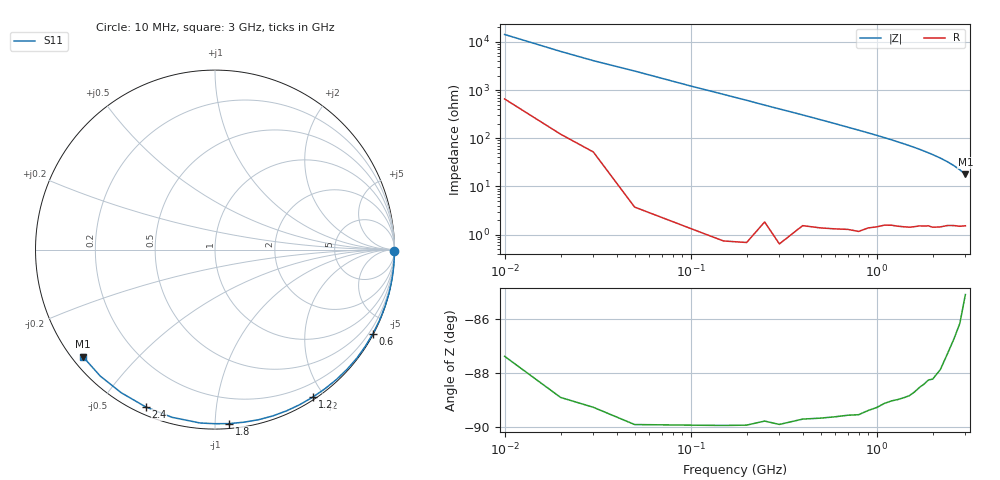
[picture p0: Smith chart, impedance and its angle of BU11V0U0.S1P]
! SIEMENS Small Signal Semiconductors
! BB833
! Si Tuning Diode in SOD323
! VR = 11 V
! S-Parameters:  April  1996
# GHz  S  MA  R  50
!  f  S11
! GHz  MAG  ANG
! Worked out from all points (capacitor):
!   31 points, 10 MHz to 3 GHz, reference 50 ohm
!   read as one part to ground: C = 1.25 pF near 10 MHz
!   lowest |Z| = 17.8 ohm at 3 GHz (marker M1)
!   S11 on the Smith chart (normalised r, x): 10 MHz: open; 600 MHz: 0.03, -4.01; 1.2 GHz: 0.03, -1.86; 1.8 GHz: 0.03, -1.08; 2.4 GHz: 0.03, -0.65; 3 GHz: 0.03, -0.35
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0.01  0.9997 -0.4
0.05  0.9999 -2.3
0.1  0.9999 -4.7
0.2  0.9998 -9.3
0.25  0.9992 -11.7
0.3  0.9996 -14.0
0.4  0.9984 -18.6
0.5  0.9978 -23.3
0.6  0.9969 -28.0
0.7  0.9959 -32.8
0.8  0.9952 -37.5
0.9  0.9929 -42.2
1  0.9909 -46.9
1.1  0.9881 -51.7
1.2  0.9861 -56.5
1.3  0.9846 -61.4
1.4  0.9829 -66.1
1.5  0.981 -70.9
1.6  0.9782 -75.7
1.7  0.975 -80.5
1.8  0.9727 -85.4
1.9  0.97 -90.2
2  0.9696 -94.9
2.2  0.9646 -104.4
2.4  0.9576 -113.8
2.6  0.9534 -123.2
2.8  0.9514 -132.2
3  0.9473 -141.0
